| IBIS file stm32u3b5_3c5_lqfp64.ibs
[IBIS ver] 4.2
[File name] stm32u3b5_3c5_lqfp64.ibs
[File Rev] 0.1
[Date] 09-03-2026
[Source] Data Created at STMicroelectronics
[Notes]  File originated from ELDO simulations.
[Disclaimer]  This information is for modeling purpose only and is
   not guaranted. The information is subject to change without
   notice.
[Copyright] Copyright 2026 STMicroelectronics Inc.
|   Component stm32u3b5_3c5_lqfp64
[Component] stm32u3b5_3c5_lqfp64
[Manufacturer] STMicroelectronics
[Package]
| variable   typ   min   max
R_pkg  0  NA  NA
L_pkg  0  NA  NA
C_pkg  0  NA  NA
[Pin]   signal_name   model_name
1  VBAT  power
2  PC13  io8_ft_100m_v33
3  PC14-OSC32_IN  io_ft_tamp
4  PC15-OSC32_OUT  io_ft_tamp
5  PH0-OSC_IN  io8_ft_100m
6  PH1-OSC_OUT  io8_ft_100m
7  NRST  ioreset_v33
8  PC0  io8_ft_100m_hslv
9  PC1  io8_ft_100m_hslv
10  PC2  io8_ft_100m_hslv
11  PC3  io8_ft_100m_hslv
12  VSSA_VREFM  nc
13  VDDA_VREFP  nc
14  PA0  io8_ft_100m
15  PA1  io8_ft_100m_hslv
16  PA2  io8_ft_100m_hslv
17  PA3  io8_ft_100m_hslv
18  VSS  gnd
19  VDD  power
20  PA4  io8_ft_100m_hslv
21  PA5  io8_ft_100m
22  PA6  io8_ft_100m_hslv
23  PA7  io8_ft_100m_hslv
24  PC4  io8_ft_100m_hslv
25  PC5  io8_ft_100m
26  PB0  io8_ft_100m_hslv
27  PB1  io8_ft_100m_hslv
28  PB2  io8_ft_100m_hslv
29  PB10  io8_ft_100m_hslv
30  VCAP  nc
31  VSS  gnd
32  VDD  power
33  PB12  io8_ft_100m_hslv
34  PB13  io8_ft_100m_hslv
35  PB14  io8_ft_100m_hslv
36  PB15  io8_ft_100m
37  PC6  io8_ft_100m_hslv
38  PC7  io8_ft_100m_hslv
39  PC8  io8_ft_100m_hslv
40  PC9  io8_ft_100m_hslv
41  PA8  io8_ft_100m_hslv
42  PA9  io8_ft_100m
43  PA10  io8_ft_100m
44  PA11  io8usb_ft_phy
45  PA12  io8usb_ft_phy
46  PA13  io8_ft_100m
47  VSS  gnd
48  VDDUSB  power
49  PA14  io8_ft_100m
50  PA15  io8_ft_100m
51  PC10  io8_ft_100m_hslv
52  PC11  io8_ft_100m_hslv
53  PC12  io8_ft_100m_hslv
54  PD2  io8_ft_100m_hslv
55  PB3  io8_ft_100m_hslv
56  PB4  io8_ft_100m_hslv
57  PB5  io8_ft_100m_hslv
58  PB6  io8_ft_100m_hslv
59  PB7  io8_ft_100m_hslv
60  PH3-BOOT0  io8_ft_100m_hslv
61  PB8  io8_ft_100m_hslv
62  PB9  io8_ft_100m_hslv
63  VSS  gnd
64  VDD  power
[Package Model]   42a-lqfp-10x10-64-251212
[Pin Mapping]   pulldown_ref   pullup_ref   | Comment
1  nc  vsw
2  gndio  vsw
3  gndio  vsw
4  gndio  vsw
5  gndio  vddio
6  gndio  vddio
7  gndio  vddio
8  gndio  vddio
9  gndio  vddio
10  gndio  vddio
11  gndio  vddio
12  nc  nc
13  nc  nc
14  gndio  vddio
15  gndio  vddio
16  gndio  vddio
17  gndio  vddio
18  gndio  nc
19  nc  vddio
20  gndio  vddio
21  gndio  vddio
22  gndio  vddio
23  gndio  vddio
24  gndio  vddio
25  gndio  vddio
26  gndio  vddio
27  gndio  vddio
28  gndio  vddio
29  gndio  vddio
30  nc  nc
31  gndio  nc
32  nc  vddio
33  gndio  vddio
34  gndio  vddio
35  gndio  vddio
36  gndio  vddio
37  gndio  vddio
38  gndio  vddio
39  gndio  vddio
40  gndio  vddio
41  gndio  vddio
42  gndio  vddio
43  gndio  vddio
44  gndio  vddusb  | Depending on IO usage
| 44  gndio  vddio  | Depending on IO usage
45  gndio  vddusb  | Depending on IO usage
| 45  gndio  vddio  | Depending on IO usage
46  gndio  vddio
47  gndio  nc
48  nc  vddusb
49  gndio  vddio
50  gndio  vddio
51  gndio  vddio
52  gndio  vddio
53  gndio  vddio
54  gndio  vddio
55  gndio  vddio
56  gndio  vddio
57  gndio  vddio
58  gndio  vddio
59  gndio  vddio
60  gndio  vddio
61  gndio  vddio
62  gndio  vddio
63  gndio  nc
64  nc  vddio
|[Diff Pin]  inv_pin  vdiff  tdelay_typ  tdelay_min  tdelay_max
|45  44  NA  NA  NA  NA
[Model Selector] io8_ft_100m
io8_ft_100m_ls_1v2  "GPIO 100MHz - 5V tolerant - low speed - 1.2V range"
io8_ft_100m_ls_1v8  "GPIO 100MHz - 5V tolerant - low speed - 1.8V range"
io8_ft_100m_ls_3v3  "GPIO 100MHz - 5V tolerant - low speed - 3.3V range"
io8_ft_100m_ms_1v2  "GPIO 100MHz - 5V tolerant - med speed - 1.2V range"
io8_ft_100m_ms_1v8  "GPIO 100MHz - 5V tolerant - med speed - 1.8V range"
io8_ft_100m_ms_3v3  "GPIO 100MHz - 5V tolerant - med speed - 3.3V range"
io8_ft_100m_fs_1v2  "GPIO 100MHz - 5V tolerant - fast speed - 1.2V range"
io8_ft_100m_fs_1v8  "GPIO 100MHz - 5V tolerant - fast speed - 1.8V range"
io8_ft_100m_fs_3v3  "GPIO 100MHz - 5V tolerant - fast speed - 3.3V range"
io8_ft_100m_hs_1v2  "GPIO 100MHz - 5V tolerant - high speed - 1.2V range"
io8_ft_100m_hs_1v8  "GPIO 100MHz - 5V tolerant - high speed - 1.8V range"
io8_ft_100m_hs_3v3  "GPIO 100MHz - 5V tolerant - high speed - 3.3V range"
[Model Selector] io8_ft_100m_hslv
io8_ft_100m_ls_1v2  "GPIO 100MHz - 5V tolerant - low speed - 1.2V range"
io8_ft_100m_ls_1v8  "GPIO 100MHz - 5V tolerant - low speed - 1.8V range"
io8_ft_100m_ls_3v3  "GPIO 100MHz - 5V tolerant - low speed - 3.3V range"
io8_ft_100m_ms_1v2  "GPIO 100MHz - 5V tolerant - med speed - 1.2V range"
io8_ft_100m_ms_1v8  "GPIO 100MHz - 5V tolerant - med speed - 1.8V range"
io8_ft_100m_ms_3v3  "GPIO 100MHz - 5V tolerant - med speed - 3.3V range"
io8_ft_100m_fs_1v2  "GPIO 100MHz - 5V tolerant - fast speed - 1.2V range"
io8_ft_100m_fs_1v8  "GPIO 100MHz - 5V tolerant - fast speed - 1.8V range"
io8_ft_100m_fs_3v3  "GPIO 100MHz - 5V tolerant - fast speed - 3.3V range"
io8_ft_100m_hs_1v2  "GPIO 100MHz - 5V tolerant - high speed - 1.2V range"
io8_ft_100m_hs_1v8  "GPIO 100MHz - 5V tolerant - high speed - 1.8V range"
io8_ft_100m_hs_3v3  "GPIO 100MHz - 5V tolerant - high speed - 3.3V range"
io8_ft_100m_hslv_ls_1v2  "GPIO 100MHz low voltage optimization - 5V tolerant - low speed - 1.2V range"
io8_ft_100m_hslv_ls_1v8  "GPIO 100MHz low voltage optimization - 5V tolerant - low speed - 1.8V range"
io8_ft_100m_hslv_ls_2v5  "GPIO 100MHz low voltage optimization - 5V tolerant - low speed - 3.3V range"
io8_ft_100m_hslv_ms_1v2  "GPIO 100MHz low voltage optimization - 5V tolerant - med speed - 1.2V range"
io8_ft_100m_hslv_ms_1v8  "GPIO 100MHz low voltage optimization - 5V tolerant - med speed - 1.8V range"
io8_ft_100m_hslv_ms_2v5  "GPIO 100MHz low voltage optimization - 5V tolerant - med speed - 3.3V range"
io8_ft_100m_hslv_fs_1v2  "GPIO 100MHz low voltage optimization - 5V tolerant - fast speed - 1.2V range"
io8_ft_100m_hslv_fs_1v8  "GPIO 100MHz low voltage optimization - 5V tolerant - fast speed - 1.8V range"
io8_ft_100m_hslv_fs_2v5  "GPIO 100MHz low voltage optimization - 5V tolerant - fast speed - 3.3V range"
io8_ft_100m_hslv_hs_1v2  "GPIO 100MHz low voltage optimization - 5V tolerant - high speed - 1.2V range"
io8_ft_100m_hslv_hs_1v8  "GPIO 100MHz low voltage optimization - 5V tolerant - high speed - 1.8V range"
io8_ft_100m_hslv_hs_2v5  "GPIO 100MHz low voltage optimization - 5V tolerant - high speed - 3.3V range"
[Model Selector] io8_ft_100m_v33
io8_ft_100m_v33_ls_1v2  "GPIO_V33 100MHz - 5V tolerant - low speed - 1.2V range"
io8_ft_100m_v33_ls_1v8  "GPIO_V33 100MHz - 5V tolerant - low speed - 1.8V range"
io8_ft_100m_v33_ls_3v3  "GPIO_V33 100MHz - 5V tolerant - low speed - 3.3V range"
io8_ft_100m_v33_ms_1v2  "GPIO_V33 100MHz - 5V tolerant - med speed - 1.2V range"
io8_ft_100m_v33_ms_1v8  "GPIO_V33 100MHz - 5V tolerant - med speed - 1.8V range"
io8_ft_100m_v33_ms_3v3  "GPIO_V33 100MHz - 5V tolerant - med speed - 3.3V range"
io8_ft_100m_v33_fs_1v2  "GPIO_V33 100MHz - 5V tolerant - fast speed - 1.2V range"
io8_ft_100m_v33_fs_1v8  "GPIO_V33 100MHz - 5V tolerant - fast speed - 1.8V range"
io8_ft_100m_v33_fs_3v3  "GPIO_V33 100MHz - 5V tolerant - fast speed - 3.3V range"
io8_ft_100m_v33_hs_1v2  "GPIO_V33 100MHz - 5V tolerant - high speed - 1.2V range"
io8_ft_100m_v33_hs_1v8  "GPIO_V33 100MHz - 5V tolerant - high speed - 1.8V range"
io8_ft_100m_v33_hs_3v3  "GPIO_V33 100MHz - 5V tolerant - high speed - 3.3V range"
[Model Selector] io8usb_ft_phy
io8_ft_100m_ls_1v2  "GPIO 100MHz - 5V tolerant - low speed - 1.2V range"
io8_ft_100m_ls_1v8  "GPIO 100MHz - 5V tolerant - low speed - 1.8V range"
io8_ft_100m_ls_3v3  "GPIO 100MHz - 5V tolerant - low speed - 3.3V range"
io8_ft_100m_ms_1v2  "GPIO 100MHz - 5V tolerant - med speed - 1.2V range"
io8_ft_100m_ms_1v8  "GPIO 100MHz - 5V tolerant - med speed - 1.8V range"
io8_ft_100m_ms_3v3  "GPIO 100MHz - 5V tolerant - med speed - 3.3V range"
io8_ft_100m_fs_1v2  "GPIO 100MHz - 5V tolerant - fast speed - 1.2V range"
io8_ft_100m_fs_1v8  "GPIO 100MHz - 5V tolerant - fast speed - 1.8V range"
io8_ft_100m_fs_3v3  "GPIO 100MHz - 5V tolerant - fast speed - 3.3V range"
io8_ft_100m_hs_1v2  "GPIO 100MHz - 5V tolerant - high speed - 1.2V range"
io8_ft_100m_hs_1v8  "GPIO 100MHz - 5V tolerant - high speed - 1.8V range"
io8_ft_100m_hs_3v3  "GPIO 100MHz - 5V tolerant - high speed - 3.3V range"
io8usb_ft_phy_hs_3v3   "USB full speed"
io8usb_ft_phy_ls_3v3   "USB low speed"
[Model Selector] io_ft_tamp
io_ft_tamp_ls_1v2 "io8_ft tamp low speed @ 1.2V"
io_ft_tamp_ls_1v8 "io8_ft tamp low speed @ 1.8V"
io_ft_tamp_ls_3v3 "io8_ft tamp low speed @ 3.3V"
io_ft_tamp_ms_1v2 "io8_ft tamp med speed @ 1.2V"
io_ft_tamp_ms_1v8 "io8_ft tamp med speed @ 1.8V"
io_ft_tamp_ms_3v3 "io8_ft tamp med speed @ 3.3V"
io_ft_tamp_fs_1v2 "io8_ft tamp fast speed @ 1.2V"
io_ft_tamp_fs_1v8 "io8_ft tamp fast speed @ 1.8V"
io_ft_tamp_fs_3v3 "io8_ft tamp fast speed @ 3.3V"
io_ft_tamp_hs_1v2 "io8_ft tamp high speed @ 1.2V"
io_ft_tamp_hs_1v8 "io8_ft tamp high speed @ 1.8V"
io_ft_tamp_hs_3v3 "io8_ft tamp high speed @ 3.3V"
[Model Selector] ioreset_v33
ioreset_v33_1v2 "Reset PAD. 5V tolerant. 1.2V range"
ioreset_v33_1v8 "Reset PAD. 5V tolerant. 1.8V range"
ioreset_v33_3v3 "Reset PAD. 5V tolerant. 3.3V range"
[Define Package Model]  42a-lqfp-10x10-64-251212
[Manufacturer]  Unknown
[OEM]  Unknown
[Description]  None
[Number Of Pins]  62
[Pin Numbers]
| Pin Num   Terminal Name
7 | NRST
14 | PA0
15 | PA1
16 | PA2
17 | PA3
20 | PA4
21 | PA5
22 | PA6
23 | PA7
41 | PA8
42 | PA9
43 | PA10
44 | PA11
45 | PA12
46 | PA13
49 | PA14
50 | PA15
26 | PB0
27 | PB1
28 | PB2
55 | PB3
56 | PB4
57 | PB5
58 | PB6
59 | PB7
61 | PB8
62 | PB9
29 | PB10
33 | PB12
34 | PB13
35 | PB14
36 | PB15
8 | PC0
9 | PC1
10 | PC2
11 | PC3
24 | PC4
25 | PC5
37 | PC6
38 | PC7
39 | PC8
40 | PC9
51 | PC10
52 | PC11
53 | PC12
2 | PC13
3 | PC14-OSC32_IN
4 | PC15-OSC32_OUT
54 | PD2
5 | PH0-OSC_IN
6 | PH1-OSC_OUT
60 | PH3-BOOT0
1 | VBAT
30 | VCAP
19 | VDD
32 | VDD
64 | VDD
13 | VDDA_VREFP
48 | VDDUSB
18 | VSS
47 | VSS
12 | VSSA_VREFM
|[Merged Pins]  18
|31  |  VSS
|63  |  VSS
[Model Data]
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[End Model Data]
[End Package Model]
|End [Component]
| Models and submodels in the file (53): io8_ft_100m_fs_1v2 (I/O), io8_ft_100m_fs_1v8 (I/O), io8_ft_100m_fs_3v3 (I/O), io8_ft_100m_hs_1v2 (I/O), io8_ft_100m_hs_1v8 (I/O), io8_ft_100m_hs_3v3 (I/O), io8_ft_100m_hslv_fs_1v2 (I/O), io8_ft_100m_hslv_fs_1v8 (I/O), io8_ft_100m_hslv_fs_2v5 (I/O), io8_ft_100m_hslv_hs_1v2 (I/O), io8_ft_100m_hslv_hs_1v8 (I/O), io8_ft_100m_hslv_hs_2v5 (I/O), io8_ft_100m_hslv_ls_1v2 (I/O), io8_ft_100m_hslv_ls_1v8 (I/O), io8_ft_100m_hslv_ls_2v5 (I/O), io8_ft_100m_hslv_ms_1v2 (I/O), io8_ft_100m_hslv_ms_1v8 (I/O), io8_ft_100m_hslv_ms_2v5 (I/O), io8_ft_100m_ls_1v2 (I/O), io8_ft_100m_ls_1v8 (I/O), io8_ft_100m_ls_3v3 (I/O), io8_ft_100m_ms_1v2 (I/O), io8_ft_100m_ms_1v8 (I/O), io8_ft_100m_ms_3v3 (I/O), io8_ft_100m_v33_fs_1v2 (I/O), io8_ft_100m_v33_fs_1v8 (I/O), io8_ft_100m_v33_fs_3v3 (I/O), io8_ft_100m_v33_hs_1v2 (I/O), io8_ft_100m_v33_hs_1v8 (I/O), io8_ft_100m_v33_hs_3v3 (I/O), io8_ft_100m_v33_ls_1v2 (I/O), io8_ft_100m_v33_ls_1v8 (I/O), io8_ft_100m_v33_ls_3v3 (I/O), io8_ft_100m_v33_ms_1v2 (I/O), io8_ft_100m_v33_ms_1v8 (I/O), io8_ft_100m_v33_ms_3v3 (I/O), io8usb_ft_phy_hs_3v3 (I/O), io8usb_ft_phy_ls_3v3 (I/O), io_ft_tamp_fs_1v2 (I/O), io_ft_tamp_fs_1v8 (I/O), io_ft_tamp_fs_3v3 (I/O), io_ft_tamp_hs_1v2 (I/O), io_ft_tamp_hs_1v8 (I/O), io_ft_tamp_hs_3v3 (I/O), io_ft_tamp_ls_1v2 (I/O), io_ft_tamp_ls_1v8 (I/O), io_ft_tamp_ls_3v3 (I/O), io_ft_tamp_ms_1v2 (I/O), io_ft_tamp_ms_1v8 (I/O), io_ft_tamp_ms_3v3 (I/O), ioreset_v33_1v2 (I/O_open_drain), ioreset_v33_1v8 (I/O_open_drain), ioreset_v33_3v3 (I/O_open_drain)
